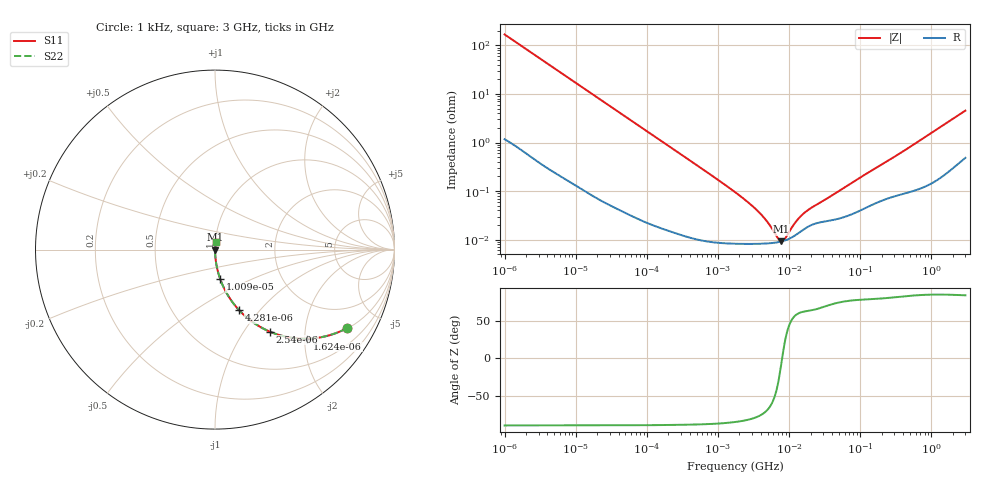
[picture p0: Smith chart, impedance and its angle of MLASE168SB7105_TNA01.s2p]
! MLASE168SB7105_TNA01  S-PARAMETER MODEL  ( Standard Model )
! Model Generated by TAIYO YUDEN Corporation (http://www.ty-top.com)
! Version 1.0
! TAIYO YUDEN Control No. 220601
! Copyright(c) 2009 TAIYO YUDEN CO.,LTD. All Rights Reserved.
! Product Description (link to TY-COMPAS)
! https://ds.yuden.co.jp/TYCOMPAS/or/detail?pn=MLASE168SB7105KTNA01&u=M
! Products Name : Multilayer Ceramic Capacitors
! Characteristics :
!  Capacitance : 1 [uF] , Rated Voltage : 16 [V] , TCC : X7R
!  Case Size : 1.6 x 0.8 / 0.063 x 0.031 [mm/inch] , Thickness : 0.8 / 0.031 [mm/inch]
!  (Conditions: Temperature = 25 [degC] , DC Bias Voltage = 0 [V])
! External Node Assignments :
!  1  o---| |---o  2
! GND o---------o GND
! Frequency Range : 1kHz  -  3GHz  [ 401 STEP ]
# MHZ S RI R 50
! Freq[MHz].  S11 Real  S11 Imag  S21 Real  S21 Imag  S12 Real  S12 Imag  S22 Real  S22 Imag
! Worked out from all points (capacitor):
!   401 points, 1 kHz to 3 GHz, reference 50 ohm
!   read as one part in series: C = 952 nF near 1.077 kHz
!   lowest |Z| = 9.29 mohm at 7.696 MHz (marker M1)
!   series resonance near 7.966 MHz, so ESL is about 420 pH
!   S11 on the Smith chart (normalised r, x): 1 kHz: 1.02, -3.34; 1.624 kHz: 1.01, -2.06; 2.54 kHz: 1.01, -1.32; 4.281 kHz: 1.01, -0.79; 10.09 kHz: 1.00, -0.33; 3 GHz: 1.01, +0.09
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0.001  0.7345 -0.4381  0.2655 0.4381  0.2655 0.4381  0.7345 -0.4381
0.001624  0.5151 -0.4962  0.4849 0.4962  0.4849 0.4962  0.5151 -0.4962
0.00254  0.3049 -0.4569  0.6951 0.4569  0.6951 0.4569  0.3049 -0.4569
0.004281  0.1353 -0.3386  0.8647 0.3386  0.8647 0.3386  0.1353 -0.3386
0.006215  0.0699 -0.2514  0.9301 0.2514  0.9301 0.2514  0.0699 -0.2514
0.010091  0.0284 -0.1622  0.9716 0.1622  0.9716 0.1622  0.0284 -0.1622
0.01216  0.02 -0.136  0.98 0.136  0.98 0.136  0.02 -0.136
0.033275  0.00306 -0.0508  0.9969 0.0508  0.9969 0.0508  0.00306 -0.0508
0.147855  0.000312 -0.0116  0.9997 0.0116  0.9997 0.0116  0.000312 -0.0116
1.732051  8.35e-05 -0.000951  0.9999 0.000951  0.9999 0.000951  8.35e-05 -0.000951
2.709407  8.22e-05 -0.000566  0.9999 0.000566  0.9999 0.000566  8.22e-05 -0.000566
3.789741  8.26e-05 -0.000355  0.9999 0.000355  0.9999 0.000355  8.26e-05 -0.000355
5.106836  8.42e-05 -0.000201  0.9999 0.000201  0.9999 0.000201  8.42e-05 -0.000201
6.881678  8.86e-05 -6.45e-05  0.9999 6.45e-05  0.9999 6.45e-05  8.86e-05 -6.45e-05
7.696136  9.16e-05 -1.51e-05  0.9999 1.51e-05  0.9999 1.51e-05  9.16e-05 -1.51e-05
8.291982  9.43e-05 1.77e-05  0.9999 -1.77e-05  0.9999 -1.77e-05  9.43e-05 1.77e-05
8.933959  9.78e-05 5.06e-05  0.9999 -5.06e-05  0.9999 -5.06e-05  9.78e-05 5.06e-05
11.59828  0.000118 0.000167  0.9999 -0.000167  0.9999 -0.000167  0.000118 0.000167
14.50609  0.000147 0.000266  0.9999 -0.000266  0.9999 -0.000266  0.000147 0.000266
21.06097  0.000204 0.000418  0.9998 -0.000418  0.9998 -0.000418  0.000204 0.000418
256.0921  0.000741 0.00433  0.9993 -0.00433  0.9993 -0.00433  0.000741 0.00433
3000  0.0068 0.0444  0.9932 -0.0444  0.9932 -0.0444  0.0068 0.0444
